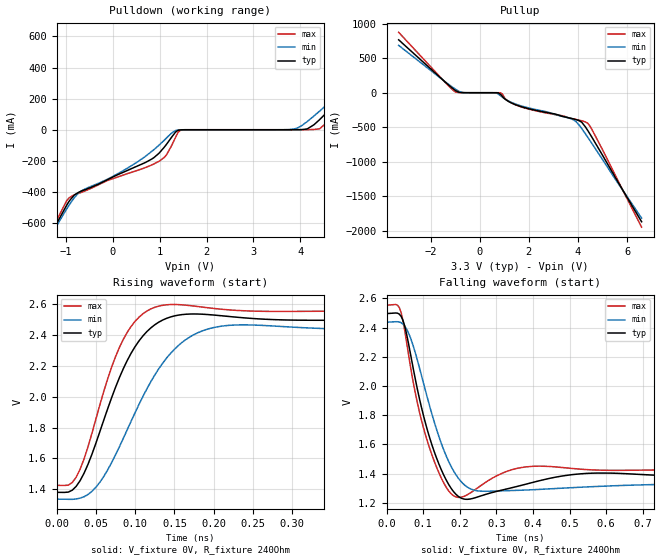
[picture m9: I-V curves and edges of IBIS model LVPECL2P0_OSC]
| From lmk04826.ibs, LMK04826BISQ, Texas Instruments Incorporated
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|   Model LVPECL2P0V
[Model]   LVPECL2P0_OSC
Model_type   Output
Polarity   Non-Inverting
Vmeas = 1.99
Vref = 1.99
Cref = .3pF
Rref = 240
|   typ   min   max
|   (nom PVT)   (fast PVT)   (slow PVT)
C_comp   0.2109p   0.1807p   0.2310p
|C_comp (Low state)   0.2109p   0.1807p   0.2310p
|C_comp (High state)   0.9933p   0.9197p   1.0724p
[Voltage Range]   3.3   3.15   3.45
[Temperature Range]   27   125   -40
[Pullup Reference]   3.3   3.15   3.45
[Pulldown Reference]   0   0   0
[Power Clamp Reference]   3.3   3.15   3.45
[GND Clamp Reference]   0   0   0
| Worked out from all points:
|   slope of the pulldown table from 0 to 0.495 V, typ, clamps not added: 7.42 ohm
|   falling waveform, V_fixture 0V, R_fixture 240Ohm: 20-80 % time 61.8ps typ, 77.5ps min, 55.1ps max; typ from 2.5 V to 1.38 V
|   rising waveform, V_fixture 0V, R_fixture 240Ohm: 20-80 % time 50.8ps typ, 66.8ps min, 42.4ps max; typ from 1.38 V to 2.5 V
[Pulldown]
|   Voltage   I(typ)   I(min)   I(max)
-3.3V     -1.869A    -1.737A    -2.051A
-1.28V    -652.5mA   -661.4mA   -639.7mA
-983.4mV  -485.5mA   -510mA     -456.6mA
-825mV    -421.3mA   -438.6mA   -419mA
986.7mV   -150.5mA   -99.33mA   -202.4mA
1.145V    -93.97mA   -53.27mA   -161.1mA
1.452V    -583uA     -287.8uA   -1.99mA
3.769V    8.124uA    1.31mA     128.1nA
4.155V    6.485mA    54.36mA    475.7uA
4.412V    65.2mA     120mA      6.277mA
5.145V    293.7mA    319.5mA    257.9mA
6.59V     761.2mA    723.2mA    811.3mA
[Pullup]
|   Voltage   I(typ)   I(min)   I(max)
-3.3V     764.4mA    683.9mA    873mA
-983.4mV  30.09mA    49.29mA    9.236mA
-686.4mV  508.5uA    3.353mA    377.6uA
561mV     -3.193uA   -260.9uA   -15.17nA
848.1mV   -23.41mA   -44.36mA   -1.6mA
1.115V    -113.3mA   -109.9mA   -110.4mA
1.531V    -182.7mA   -172.8mA   -185.6mA
3.739V    -372.4mA   -379.6mA   -372.9mA
4.125V    -420.2mA   -504.9mA   -403.5mA
4.392V    -543.2mA   -640.9mA   -440.5mA
4.966V    -883.9mA   -948.6mA   -801.6mA
6.59V     -1.865A    -1.813A    -1.943A
[Ramp]
R_load = 240
|   typ   min   max
dV/dt_r   0.669407/5.08194e-11   0.660633/6.67586e-11   0.676564/4.24188e-11
dV/dt_f   0.66946/6.18152e-11   0.660583/7.75013e-11   0.676594/5.50565e-11
[Falling Waveform]
V_fixture = 0V
V_fixture_min = 0V
V_fixture_max = 0V
R_fixture = 240Ohm
C_fixture = 0F
|   Time   V(typ)   V(min)   V(max)
0s        2.496V     2.437V     2.553V
35ps      2.492V     2.439V     2.537V
60ps      2.291V     2.364V     2.217V
85ps      1.97V      2.171V     1.877V
120ps     1.628V     1.843V     1.557V
190ps     1.258V     1.391V     1.24V
245ps     1.237V     1.284V     1.296V
400ps     1.34V      1.29V      1.45V
575ps     1.404V     1.312V     1.424V
1.9ns     1.38V      1.336V     1.426V
[Rising Waveform]
V_fixture = 0V
V_fixture_min = 0V
V_fixture_max = 0V
R_fixture = 240Ohm
C_fixture = 0F
|   Time   V(typ)   V(min)   V(max)
0s        1.381V     1.336V     1.426V
25ps      1.42V      1.338V     1.479V
55ps      1.772V     1.445V     1.944V
75ps      2.06V      1.623V     2.258V
95ps      2.282V     1.842V     2.456V
115ps     2.422V     2.051V     2.554V
140ps     2.507V     2.25V      2.595V
180ps     2.535V     2.414V     2.583V
230ps     2.514V     2.464V     2.558V
1.9ns     2.496V     2.437V     2.554V
